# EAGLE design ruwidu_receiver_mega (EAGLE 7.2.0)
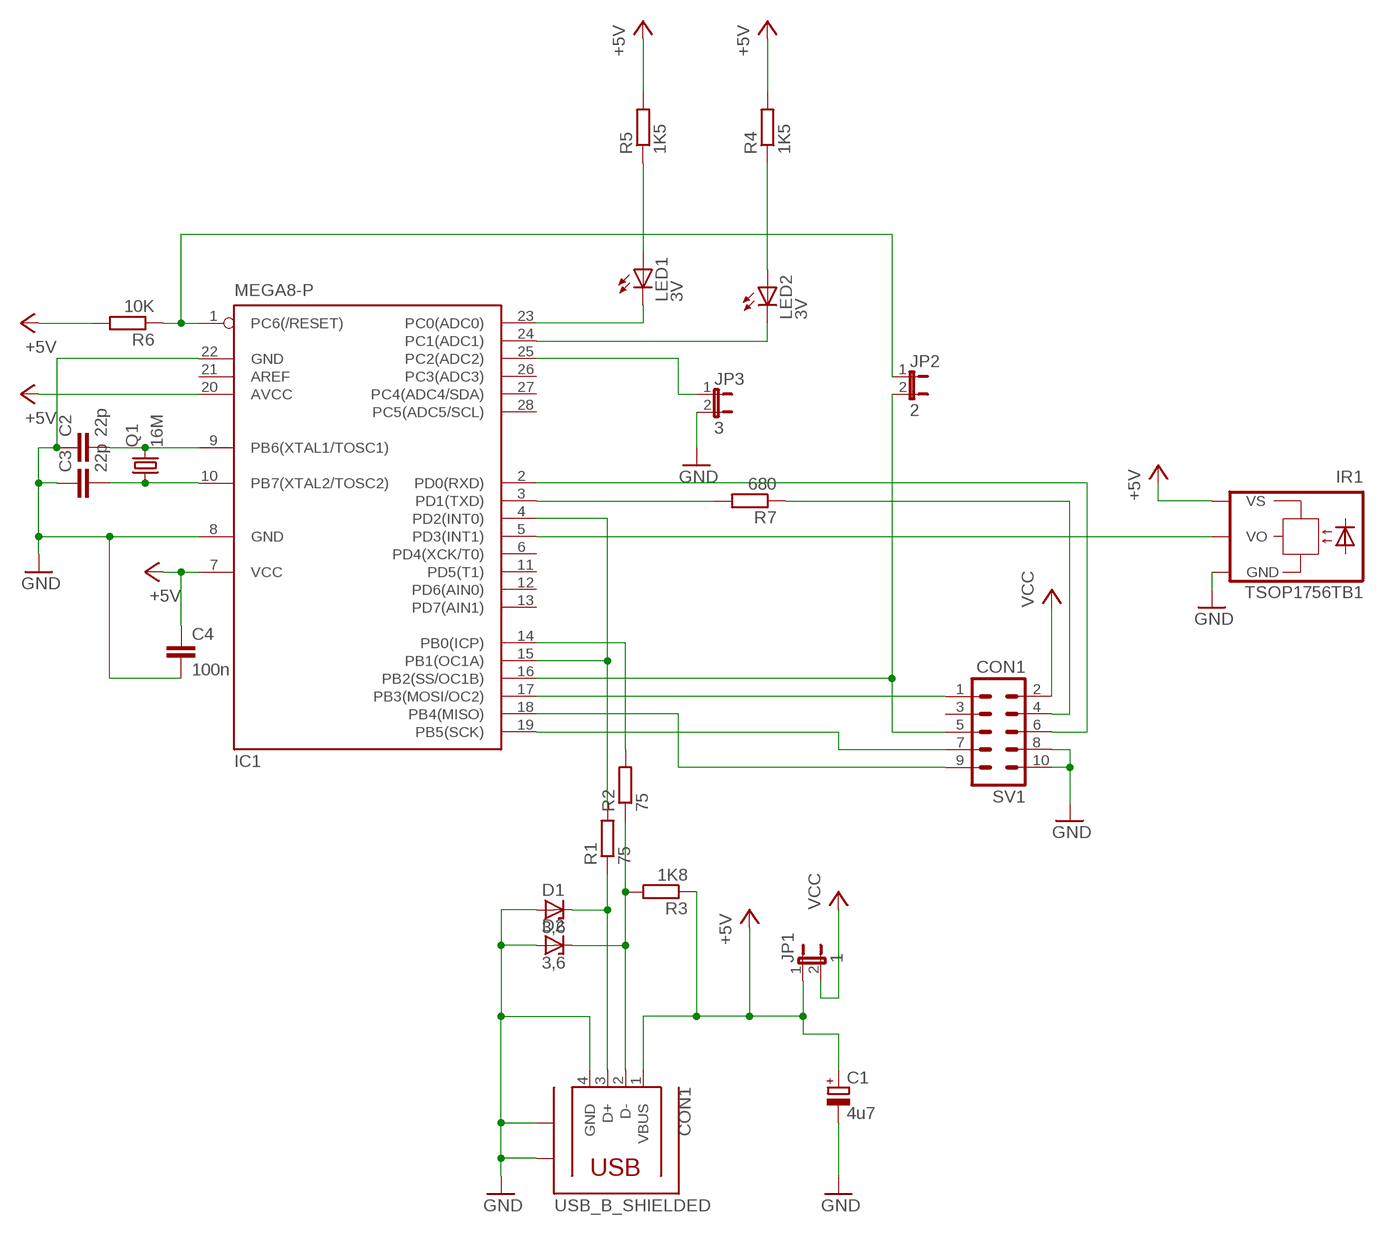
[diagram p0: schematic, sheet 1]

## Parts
C1  4u7  CPOL-EUE2-5  [E2-5]
C2  22p  C-EU025-024X044  [C025-024X044]
C3  22p  C-EU025-024X044  [C025-024X044]
C4  100n  C2,5-3  [C2.5-3]
CON1  USB_B_SHIELDED  [USB_B_SHIELDED_THMD]
D1  3,6  ZENER-DIODEDO35Z10  [DO35Z10]
D2  3,6  ZENER-DIODEDO35Z10  [DO35Z10]
IC1  MEGA8-P  [DIL28-3]
IR1  TSOP1756TB1  [TSOP17_TB1]
JP1  1  JP1E  [JP1]
JP2  2  JP1E  [JP1]
JP3  3  JP1E  [JP1]
LED1  3V  LED5MM  [LED5MM]
LED2  3V  LED5MM  [LED5MM]
Q1  16M  CRYSTALHC49S  [HC49/S]
R1  75  R-EU_0207/10  [0207/10]
R2  75  R-EU_0207/10  [0207/10]
R3  1K8  R-EU_0207/10  [0207/10]
R4  1K5  R-EU_0207/10  [0207/10]
R5  1K5  R-EU_0207/10  [0207/10]
R6  10K  R-EU_0207/10  [0207/10]
R7  680  R-EU_0207/10  [0207/10]
SV1  CON1  ML10  [ML10]

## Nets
+5V: C1.+ C4.1 CON1.1(VBUS) IC1.7(VCC) IC1.20(AVCC) IR1.VS JP1.1 R3.1 R4.2 R5.2 R6.2
GND: C1.- C2.1 C3.1 C4.2 CON1.4(GND) CON1.S1 CON1.S2 D1.A D2.A IC1.8(GND) IC1.22(GND) IR1.GND JP3.2 SV1.8 SV1.10
N$1: IC1.4(PD2(INT0)) IC1.15(PB1(OC1A)) R1.2
N$2: CON1.3(D+) D1.C R1.1
N$3: CON1.2(D-) D2.C R2.1 R3.2
N$4: IC1.14(PB0(ICP)) R2.2
N$5: IC1.17(PB3(MOSI/OC2)) SV1.1
N$6: IC1.18(PB4(MISO)) SV1.9
N$7: IC1.19(PB5(SCK)) SV1.7
N$8: IC1.1(PC6(/RESET)) JP2.1 R6.1
N$9: R7.1 SV1.4
N$10: IC1.2(PD0(RXD)) SV1.6
N$11: C2.2 IC1.9(PB6(XTAL1/TOSC1)) Q1.2
N$12: C3.2 IC1.10(PB7(XTAL2/TOSC2)) Q1.1
N$13: LED1.A R5.1
N$14: LED2.A R4.1
N$15: IC1.23(PC0(ADC0)) LED1.K(C)
N$16: IC1.24(PC1(ADC1)) LED2.K(C)
N$17: IC1.16(PB2(SS/OC1B)) JP2.2 SV1.5
N$18: IC1.25(PC2(ADC2)) JP3.1
N$19: IC1.3(PD1(TXD)) R7.2
N$20: IC1.5(PD3(INT1)) IR1.VO
VCC: JP1.2 SV1.2
Unconnected: IC1.6(PD4(XCK/T0)) IC1.11(PD5(T1)) IC1.12(PD6(AIN0)) IC1.13(PD7(AIN1)) IC1.21(AREF) IC1.26(PC3(ADC3)) IC1.27(PC4(ADC4/SDA)) IC1.28(PC5(ADC5/SCL)) SV1.3

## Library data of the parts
C1 = rcl:CPOL-EU: POLARIZED CAPACITOR, European symbol
C2 C3 = resistor:C-EU: CAPACITOR, European symbol
C4 = capacitor-wima:C: CAPACITOR
CON1 = USB:USB_B_SHIELDED
D1 D2 = diode:ZENER-DIODE: Z-Diode
IC1 = atmel:MEGA8-P: MICROCONTROLLER 8 Kbytes FLASH, 1 kbytes SRAM, 512 bytes EEPROM, USART, 4-channel 10 bit ADC, 2-channel 8 bit ADC Pin compatible with Atmega48, ATMega88, ATMega168 Source: avr.lbr
IR1 = telefunken:TSOP17*TB1: TSOP17..TB1 IR Receiver Modules for Remote Control Systems Source: http://www.vishay.com/docs/82042/82042.pdf; OC_FARNELL: unknown; OC_NEWARK: unknown
JP1-JP3 = jumper:JP1E: JUMPER
LED1 LED2 = led:LED: LED
Q1 = crystal:CRYSTAL: CRYSTAL
R1-R7 = resistor:R-EU_: RESISTOR, European symbol
SV1 = con-harting-ml:ML10: HARTING

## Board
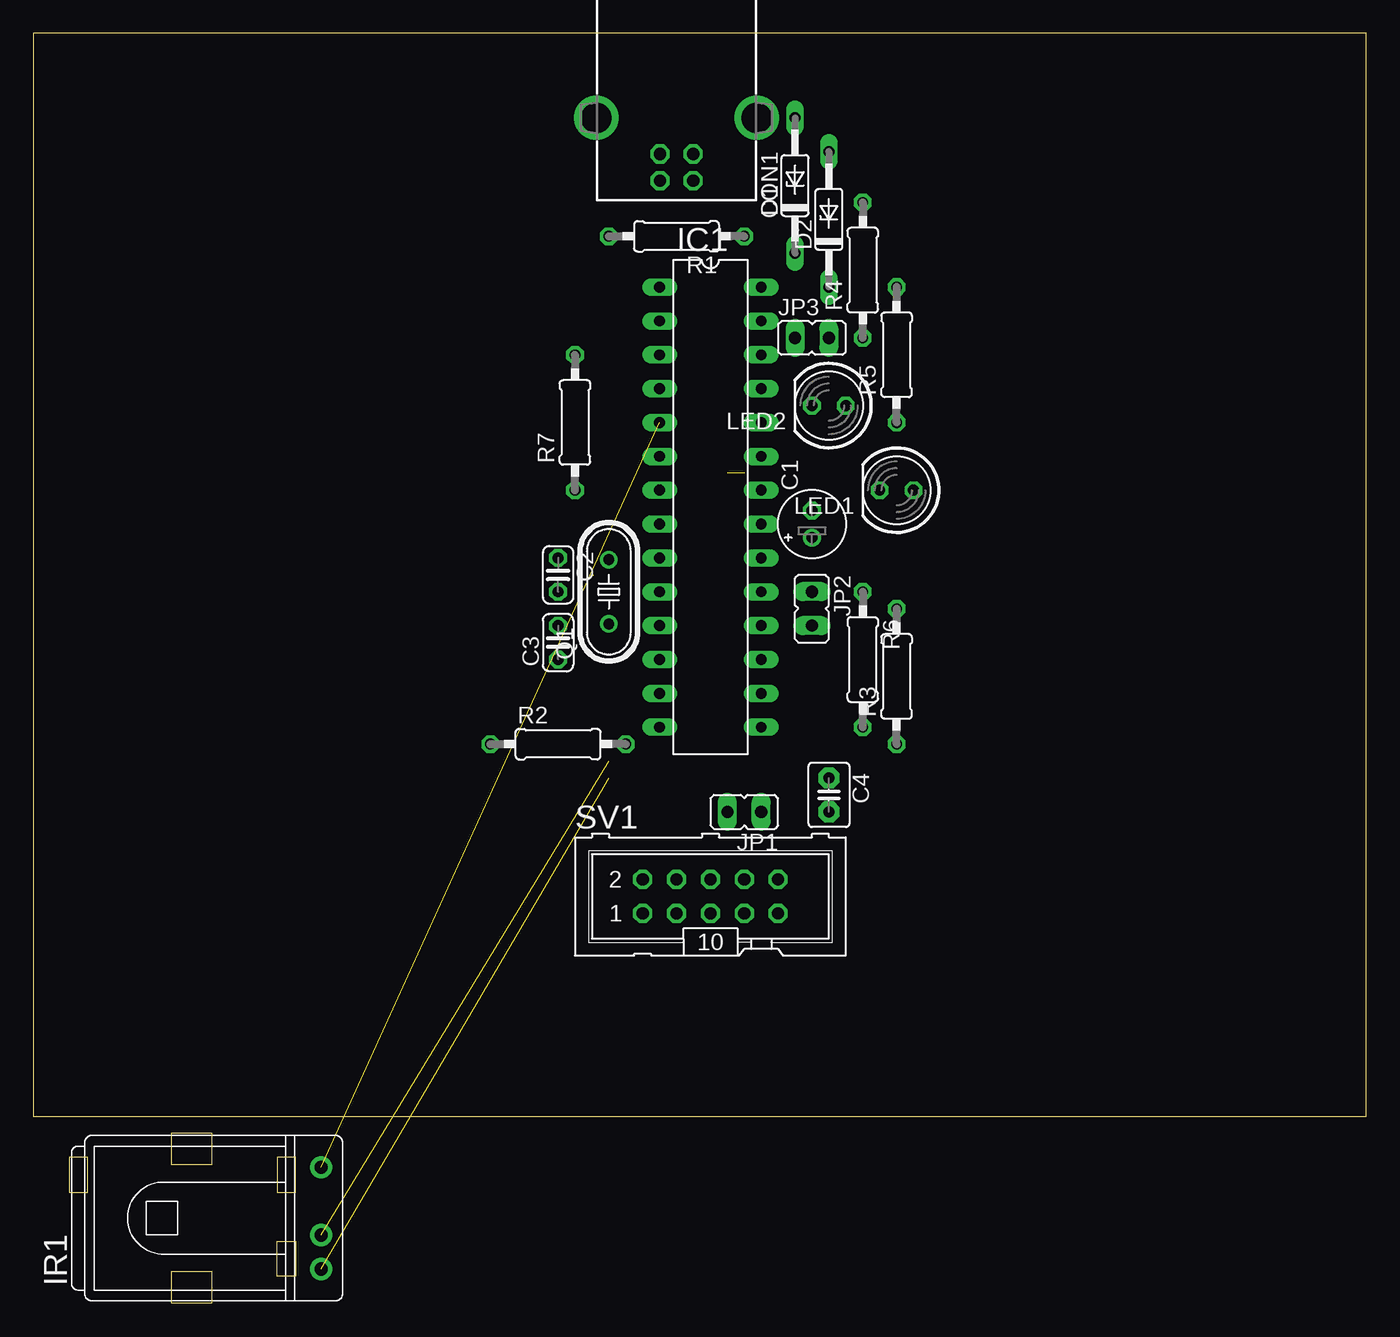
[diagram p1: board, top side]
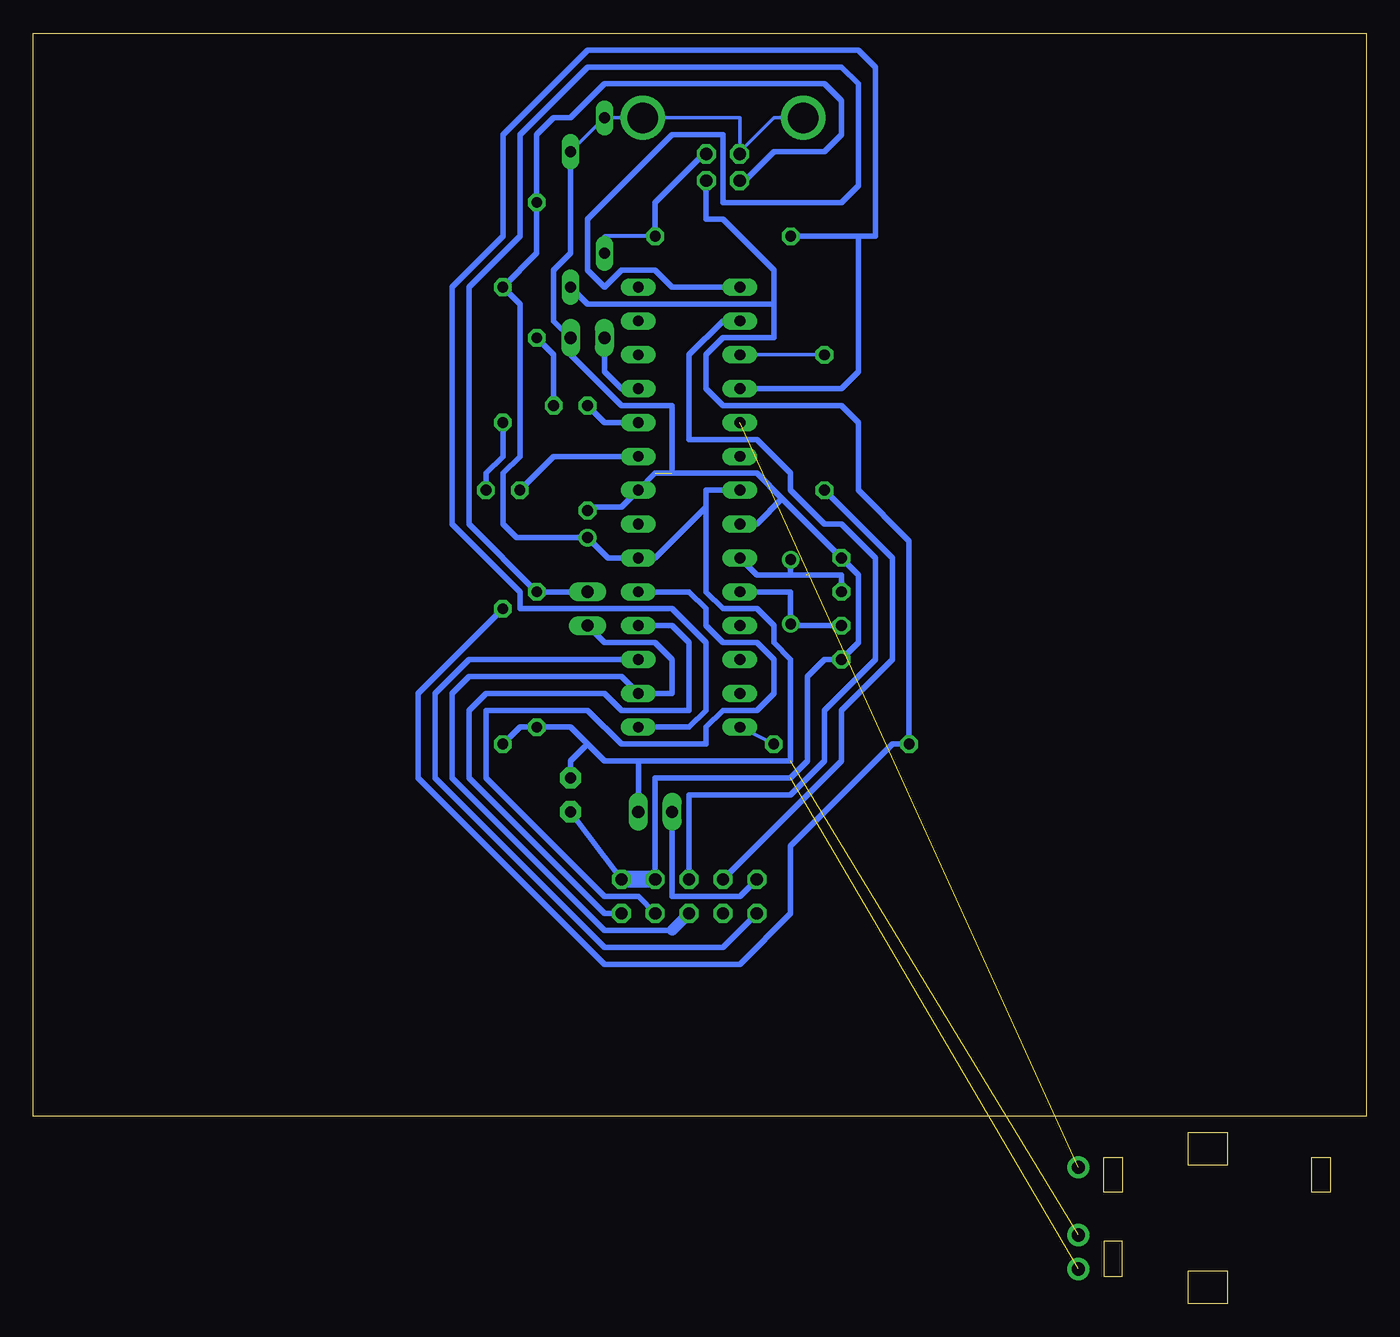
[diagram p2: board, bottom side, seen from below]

Size 100 x 95.29 mm. Coordinates in mm from the lower left corner, seen from the top.
Outline: 0,14.02 100,14.02 100,95.29 0,95.29 0,14.02
Copper layers (1*16): Top 0.035mm / dielectric 1.5mm / Bottom 0.035mm
Design rules "default": minimum track width 10mil, minimum drill 24mil, track to track 8mil, track to pad 8mil, pad to pad 8mil, via to via 8mil, smd to smd 8mil, copper to edge 40mil, drill to drill 8mil, minimum pad ring 10mil, minimum via ring 8mil, stop-mask expansion 4mil, vias tented up to drill 0mil, thermal gap 10mil

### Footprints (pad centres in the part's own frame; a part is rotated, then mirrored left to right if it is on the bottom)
E2-5 = drill 0.813 pad 1.27: + -1.016,0 | drill 0.813 pad 1.27 octagon: - 1.016,0
C025-024X044 = drill 0.813 octagon: 1 -1.27,0; 2 1.27,0
C2.5-3 = drill 0.813 pad 1.6 octagon: 1 -1.27,0; 2 1.27,0
USB_B_SHIELDED_THMD = drill 0.92 octagon: 1 4.71,-1.25; 2 4.71,1.25; 3 2.71,1.25; 4 2.71,-1.25 | drill 2.3: S1 0,6.02; S2 0,-6.02
DO35Z10 = drill 0.813 long: A 5.08,0; C -5.08,0
DIL28-3 = drill 0.813 long: 1 -16.51,-3.81; 2 -13.97,-3.81; 3 -11.43,-3.81; 4 -8.89,-3.81; 5 -6.35,-3.81; 6 -3.81,-3.81; 7 -1.27,-3.81; 8 1.27,-3.81; 9 3.81,-3.81; 10 6.35,-3.81; 11 8.89,-3.81; 12 11.43,-3.81; 13 13.97,-3.81; 14 16.51,-3.81; 15 16.51,3.81; 16 13.97,3.81; 17 11.43,3.81; 18 8.89,3.81; 19 6.35,3.81; 20 3.81,3.81; 21 1.27,3.81; 22 -1.27,3.81; 23 -3.81,3.81; 24 -6.35,3.81; 25 -8.89,3.81; 26 -11.43,3.81; 27 -13.97,3.81; 28 -16.51,3.81
TSOP17_TB1 = drill 1 pad 1.676: GND 0,-3.81; VO 0,3.81; VS 0,-1.27
JP1 = drill 0.914 long: 1 0,-1.27; 2 0,1.27
LED5MM = drill 0.813 octagon: A -1.27,0; K 1.27,0
HC49/S = drill 0.813: 1 -2.413,0; 2 2.413,0
0207/10 = drill 0.813 octagon: 1 -5.08,0; 2 5.08,0
ML10 = drill 0.914 octagon: 1 -5.08,-1.27; 2 -5.08,1.27; 3 -2.54,-1.27; 4 -2.54,1.27; 5 0,-1.27; 6 0,1.27; 7 2.54,-1.27; 8 2.54,1.27; 9 5.08,-1.27; 10 5.08,1.27

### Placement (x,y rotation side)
C1  58.42,58.47 90 top
C2  39.37,54.66 270 top
C3  39.37,49.58 90 top
C4  59.69,38.15 270 top
CON1  48.26,88.95 270 top
D1  57.15,83.87 90 top
D2  59.69,81.33 90 top
IC1  50.8,59.74 270 top
IR1  21.59,6.4 0 top
JP1  53.34,36.88 90 top
JP2  58.42,52.12 180 top
JP3  58.42,72.44 270 top
LED1  64.77,61.01 180 top
LED2  59.69,67.36 180 top
Q1  43.18,53.39 90 top
R1  48.26,80.06 180 top
R2  39.37,41.96 0 top
R3  64.77,47.04 90 top
R4  62.23,77.52 90 top
R5  64.77,71.17 90 top
R6  62.23,48.31 270 top
R7  40.64,66.09 90 top
SV1  50.8,30.53 0 top

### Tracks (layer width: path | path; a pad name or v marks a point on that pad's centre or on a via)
+5V  (1 unrouted)
  Bottom 0.254: 46.99,83.87 CON1.1
  Bottom 0.406: 49.53,59.74 49.53,53.39 48.26,52.12 45.72,52.12 44.45,50.85 44.45,49.58 43.18,48.31 43.18,40.69 54.61,40.69 | C4.1 59.69,40.69 58.42,41.96 | 58.42,41.96 57.15,40.69 54.61,40.69 | 58.42,41.96 59.69,43.23 R6.2 63.5,43.23 R3.1 | 54.61,40.69 JP1.1 | 46.99,83.87 44.45,86.41 40.64,86.41 39.37,87.68 39.37,90.22 40.64,91.49 57.15,91.49 59.69,88.95 60.96,88.95 62.23,87.68 R4.2 62.23,78.79 R5.2 63.5,74.98 63.5,63.55 64.77,62.28 64.77,58.47 63.75,57.45 C1.+ 56.9,55.93 IC1.20 53.34,55.93 49.53,59.74 | IC1.7 49.53,61.01 49.53,59.74
GND  (2 unrouted)
  Bottom 0.254: 46.99,86.41 44.45,88.95 CON1.S2 | D2.A D1.A CON1.S1 46.99,88.95 46.99,86.41 | 46.99,86.41 CON1.4
  Bottom 0.406: 52.07,62.28 52.07,67.36 55.88,67.36 59.69,71.17 JP3.2 60.96,73.71 60.96,77.52 59.69,78.79 D2.A | SV1.10 C4.2 | SV1.8 53.34,39.42 43.18,39.42 41.91,40.69 41.91,47.04 40.64,48.31 C3.1 38.1,49.58 38.1,54.66 C2.1 43.81,60.38 | C1.- 58.17,59.74 55.88,59.74 IC1.22 53.34,62.28 45.72,62.28 43.81,60.38 | IC1.8 45.72,58.47 43.81,60.38
  Bottom 1.27: SV1.8 SV1.10
N$1
  Bottom 0.254: IC1.15 53.34,43.23
  Bottom 0.406: IC1.15 50.8,43.23 49.53,44.5 49.53,49.58 52.07,52.12 63.5,52.12 63.5,53.39 68.58,58.47 68.58,76.25 64.77,80.06 64.77,87.68 58.42,94.03 38.1,94.03 36.83,92.76 36.83,80.06 38.1,80.06 | 38.1,80.06 R1.2 | 38.1,80.06 38.1,69.9 39.37,68.63 IC1.4
N$2
  Bottom 0.254: 57.15,80.06 D1.C | 49.53,86.41 CON1.3
  Bottom 0.305: R1.1 57.15,80.06
  Bottom 0.406: 49.53,86.41 53.34,82.6 R1.1
N$3
  Bottom 0.254: 49.53,83.87 CON1.2
  Bottom 0.406: CON1.2 49.53,84.22 | R3.2 71.12,45.77 71.12,39.42 57.15,25.45 46.99,25.45 43.18,29.26 43.18,34.34 35.56,41.96 R2.1 34.29,57.2 38.1,61.01 38.1,66.09 39.37,67.36 48.26,67.36 49.53,68.63 49.53,71.17 48.26,72.44 44.45,72.44 44.45,74.98 | 44.45,74.98 58.42,74.98 D2.C | 49.53,83.87 49.53,81.33 48.26,81.33 44.45,77.52 44.45,74.98
N$4
  Bottom 0.254: R2.2 IC1.14
N$5
  Bottom 0.406: IC1.17 67.31,48.31 69.85,45.77 69.85,39.42 57.15,26.72 48.26,26.72 SV1.1
N$6
  Bottom 0.406: IC1.18 52.07,50.85 50.8,49.58 50.8,44.5 55.88,44.5 57.15,45.77 66.04,45.77 67.31,44.5 67.31,39.42 57.15,29.26 SV1.9
N$7
  Bottom 0.406: SV1.7 54.61,30.53 57.15,30.53 66.04,39.42 66.04,44.5 58.42,44.5 55.88,41.96 49.53,41.96 49.53,43.23 48.26,44.5 45.72,44.5 44.45,45.77 44.45,48.31 45.72,49.58 48.26,49.58 49.53,50.85 49.53,52.12 50.8,53.39 IC1.19
N$8
  Bottom 0.406: JP2.1 R6.1 67.31,58.47 67.31,76.25 63.5,80.06 63.5,87.68 58.42,92.76 39.37,92.76 38.1,91.49 38.1,83.87 39.37,82.6 48.26,82.6 48.26,87.68 52.07,87.68 58.42,81.33 58.42,77.52 57.15,76.25 55.88,77.52 53.34,77.52 52.07,76.25 IC1.1
N$9
  Bottom 0.406: SV1.4 39.37,40.69 39.37,44.5 35.56,48.31 35.56,55.93 R7.1
N$10
  Bottom 0.406: IC1.2 48.26,73.71 50.8,71.17 50.8,64.82 45.72,64.82 43.18,62.28 43.18,61.01 40.64,58.47 39.37,58.47 36.83,55.93 36.83,48.31 40.64,44.5 40.64,40.69 43.18,38.15 50.8,38.15 SV1.6
N$11  (1 unrouted)
  Bottom 0.406: IC1.9 45.72,54.66 43.18,54.66 | 42.04,54.66 43.18,54.66 | 41.91,54.66 39.37,54.66 C2.2 | 43.18,54.66 Q1.2
N$12
  Bottom 0.406: C3.2 43.18,50.85 Q1.1 43.18,53.39 IC1.10
N$13
  Bottom 0.406: LED1.A 66.04,62.28 64.77,63.55 R5.1
N$14
  Bottom 0.406: R4.1 60.96,71.17 LED2.A
N$15
  Bottom 0.406: LED1.K 60.96,63.55 IC1.23
N$16
  Bottom 0.406: IC1.24 57.15,66.09 LED2.K
N$17
  Bottom 0.406: JP2.2 57.15,49.58 53.34,49.58 52.07,48.31 52.07,45.77 IC1.16 55.88,47.04 67.31,47.04 68.58,45.77 68.58,39.42 57.15,27.99 52.07,27.99
  Bottom 0.813: SV1.5 52.07,27.99
N$18
  Bottom 0.406: JP3.1 57.15,69.9 55.88,68.63 IC1.25
N$19
  Bottom 0.254: R7.2 IC1.3
N$20  (1 unrouted)
VCC
  Bottom 0.406: SV1.2 46.99,30.53 52.07,30.53 JP1.2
